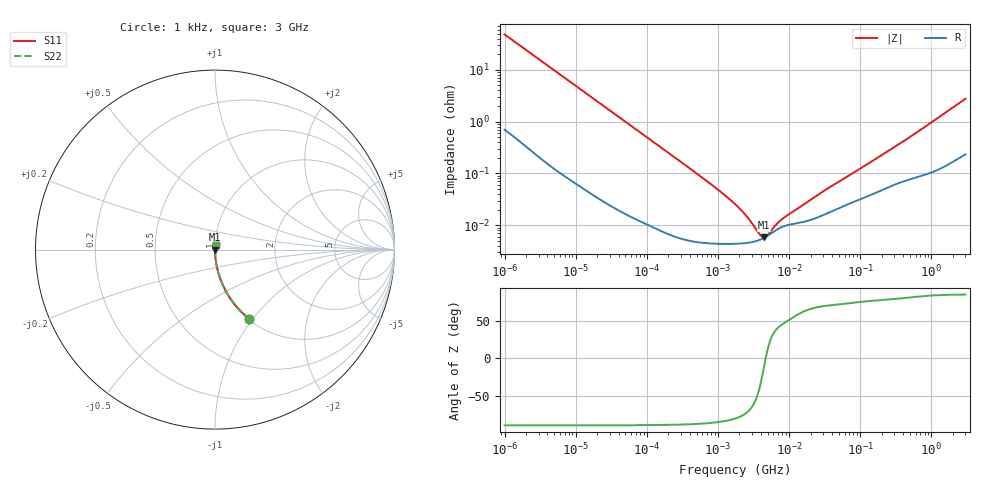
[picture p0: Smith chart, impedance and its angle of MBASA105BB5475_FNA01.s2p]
! MBASA105BB5475_FNA01  S-PARAMETER MODEL  ( Standard Model )
! Model Generated by TAIYO YUDEN Corporation (http://www.ty-top.com)
! Version 1.0
! TAIYO YUDEN Control No. 220601
! Copyright(c) 2013 TAIYO YUDEN CO.,LTD. All Rights Reserved.
! Product Description (link to TY-COMPAS)
! https://ds.yuden.co.jp/TYCOMPAS/or/detail?pn=MBASA105BB5475MFNA01&u=M
! Products Name : Multilayer Ceramic Capacitors
! Characteristics :
!  Capacitance : 4.7 [uF] , Rated Voltage : 4 [V] , TCC : X5R
!  Case Size : 1.0 x 0.5 / 0.039 x 0.02 [mm/inch] , Thickness : 0.5 / 0.02 [mm/inch]
!  (Conditions: Temperature = 25 [degC] , DC Bias Voltage = 0 [V])
! External Node Assignments :
!  1  o---| |---o  2
! GND o---------o GND
! Frequency Range : 1kHz  -  3GHz  [ 401 STEP ]
# MHZ S RI R 50
! Freq[MHz].  S11 Real  S11 Imag  S21 Real  S21 Imag  S12 Real  S12 Imag  S22 Real  S22 Imag
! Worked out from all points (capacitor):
!   401 points, 1 kHz to 3 GHz, reference 50 ohm
!   read as one part in series: C = 3.29 uF near 1.077 kHz
!   lowest |Z| = 5.81 mohm at 4.399 MHz (marker M1)
!   series resonance near 4.671 MHz, so ESL is about 350 pH
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0.001  0.1917 -0.3865  0.8083 0.3865  0.8083 0.3865  0.1917 -0.3865
0.001564  0.0906 -0.2801  0.9094 0.2801  0.9094 0.2801  0.0906 -0.2801
0.002447  0.0403 -0.19  0.9597 0.19  0.9597 0.19  0.0403 -0.19
0.004969  0.0108 -0.0971  0.9892 0.0971  0.9892 0.0971  0.0108 -0.0971
0.01216  0.00216 -0.0403  0.9978 0.0403  0.9978 0.0403  0.00216 -0.0403
0.033275  0.000444 -0.0149  0.9996 0.0149  0.9996 0.0149  0.000444 -0.0149
0.147855  9.2e-05 -0.00339  0.9999 0.00339  0.9999 0.00339  9.2e-05 -0.00339
0.762639  4.5e-05 -0.000646  1 0.000646  1 0.000646  4.5e-05 -0.000646
1.238299  4.37e-05 -0.00038  1 0.00038  1 0.00038  4.37e-05 -0.00038
1.732051  4.39e-05 -0.000253  1 0.000253  1 0.000253  4.39e-05 -0.000253
2.24859  4.47e-05 -0.000173  1 0.000173  1 0.000173  4.47e-05 -0.000173
3.14518  4.79e-05 -8.78e-05  1 8.78e-05  1 8.78e-05  4.79e-05 -8.78e-05
3.388684  4.91e-05 -7.04e-05  1 7.04e-05  1 7.04e-05  4.91e-05 -7.04e-05
4.399271  5.67e-05 -1.26e-05  0.9999 1.26e-05  0.9999 1.26e-05  5.67e-05 -1.26e-05
5.928204  7.35e-05 4.66e-05  0.9999 -4.66e-05  0.9999 -4.66e-05  7.35e-05 4.66e-05
6.387174  7.87e-05 5.95e-05  0.9999 -5.95e-05  0.9999 -5.95e-05  7.87e-05 5.95e-05
8.933959  9.84e-05 0.000111  0.9999 -0.000111  0.9999 -0.000111  9.84e-05 0.000111
21.06097  0.00013 0.000299  0.9999 -0.000299  0.9999 -0.000299  0.00013 0.000299
256.0921  0.00056 0.00274  0.9994 -0.00274  0.9994 -0.00274  0.00056 0.00274
581.6181  0.00085 0.00575  0.9992 -0.00575  0.9992 -0.00575  0.00085 0.00575
2784.426  0.00285 0.0255  0.9972 -0.0255  0.9972 -0.0255  0.00285 0.0255
3000  0.00308 0.0273  0.9969 -0.0273  0.9969 -0.0273  0.00308 0.0273
